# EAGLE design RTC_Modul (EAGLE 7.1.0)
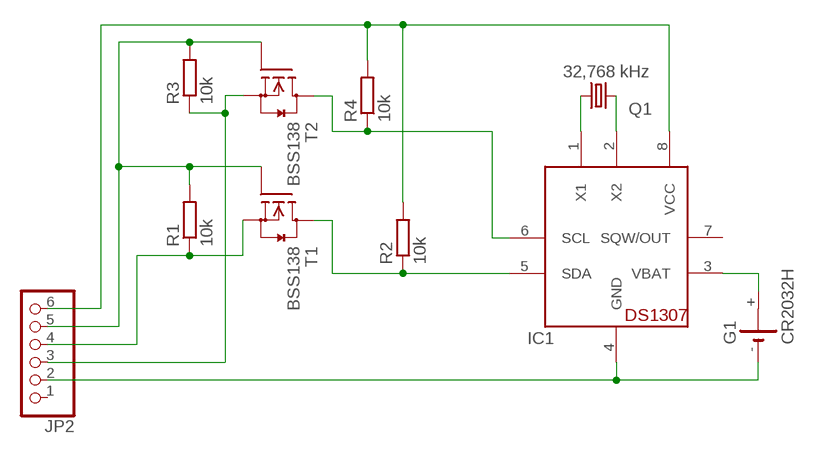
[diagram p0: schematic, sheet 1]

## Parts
G1  CR2032H  [CR2032H]
IC1  DS1307  [DIL08]
JP2  PINHD-1X6/90  [1X06/90]
Q1  32,768 kHz  CRYSTALTC26H  [TC26H]
R1  10k  R-EU_M1206  [M1206]
R2  10k  R-EU_M1206  [M1206]
R3  10k  R-EU_M1206  [M1206]
R4  10k  R-EU_M1206  [M1206]
T1  BSS138  [SOT23]
T2  BSS138  [SOT23]

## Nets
GND: G1.- IC1.4(GND) JP2.2
N$1: IC1.1(X1) Q1.1
N$2: IC1.2(X2) Q1.2
N$3: JP2.4 R1.1 T1.2(S)
N$5: G1.+ IC1.3(VBAT)
N$7: IC1.5(SDA) R2.1 T1.3(D)
N$9: JP2.3 R3.1 T2.2(S)
N$10: JP2.5 R1.2 R3.2 T1.1(G) T2.1(G)
N$11: IC1.6(SCL) R4.1 T2.3(D)
VCC: IC1.8(VCC) JP2.6 R2.2 R4.2
Unconnected: G1.+@1(+) IC1.7(SQW/OUT) JP2.1

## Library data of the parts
G1 = battery:CR2032H: LI BATTERY Varta
IC1 = adafruit:DS1307: DS1307 Real time clock (RTC) with battery backup ability. Talk to it via i2c
JP2 = pinhead:PINHD-1X6: PIN HEADER
Q1 = crystal:CRYSTAL: CRYSTAL; OC_FARNELL: unknown; OC_NEWARK: unknown
R1-R4 = rcl:R-EU_: RESISTOR, European symbol
T1 T2 = m-pad-2.1:BSS138: Fairchild Semiconductors BSS138 N-Channel Logic Level Enhancement Mode Field Effect Transistor General Description: These N-Channel enhancement mode field effect transistors are produced using Fairchild's proprietary, high cell density, DMOS technology. These products have been designed to minimize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

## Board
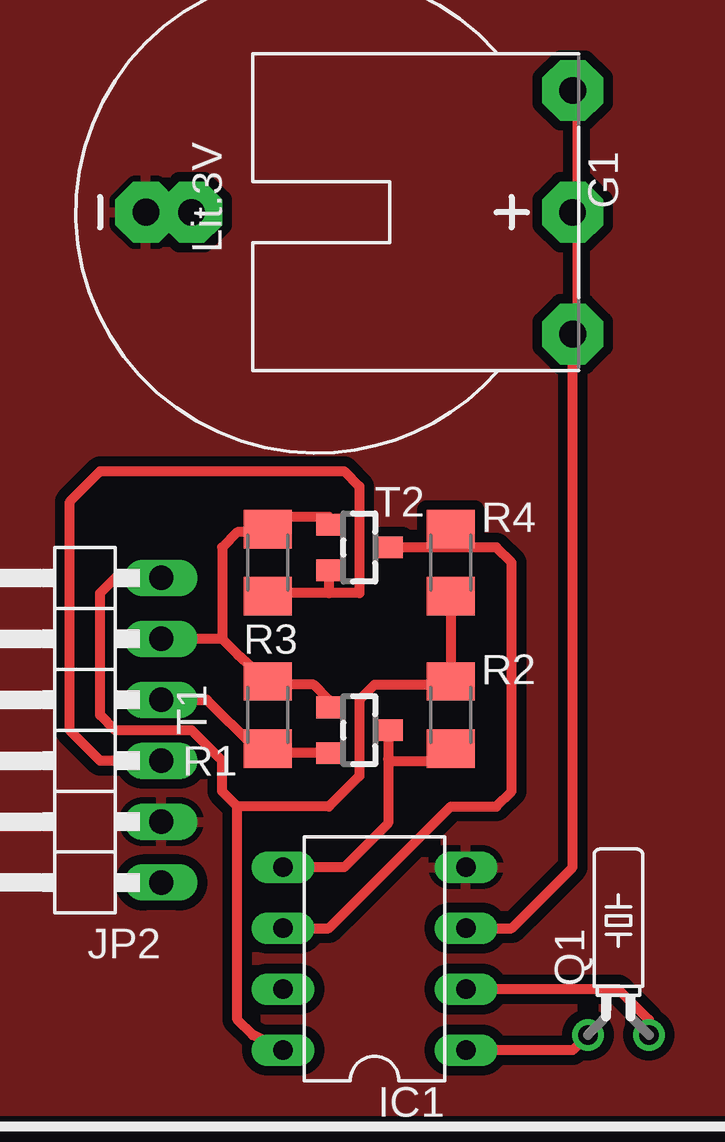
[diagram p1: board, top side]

No outline drawn. Coordinates in mm, seen from the top.
Copper layers (1*16): Top 0.035mm / dielectric 1.5mm / Bottom 0.035mm
Design rules "default": minimum track width 10mil, minimum drill 24mil, track to track 8mil, track to pad 8mil, pad to pad 8mil, via to via 8mil, smd to smd 8mil, copper to edge 40mil, drill to drill 8mil, minimum pad ring 10mil, minimum via ring 8mil, stop-mask expansion 4mil, vias tented up to drill 0mil, thermal gap 10mil

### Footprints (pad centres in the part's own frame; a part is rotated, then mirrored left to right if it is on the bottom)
CR2032H = drill 1.118 pad 2.54 octagon: + 5.08,10.795; +@1 -5.08,10.795; - 0,-6.985
DIL08 = drill 0.813 long: 1 -3.81,-3.81; 2 -1.27,-3.81; 3 1.27,-3.81; 4 3.81,-3.81; 5 3.81,3.81; 6 1.27,3.81; 7 -1.27,3.81; 8 -3.81,3.81
1X06/90 = drill 1.016 long: 1 -6.35,-3.81; 2 -3.81,-3.81; 3 -1.27,-3.81; 4 1.27,-3.81; 5 3.81,-3.81; 6 6.35,-3.81
TC26H = drill 0.813: 1 -1.27,0; 2 1.27,0
M1206 = smd 1.6 x 2: 1 -1.4,0; 2 1.4,0
SOT23 = smd 0.9 x 1.2: 1 -0.95,-1.2; 2 0.95,-1.2; 3 0,1.2

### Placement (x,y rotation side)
G1  17.78,38.1 270 top
IC1  20.32,6.99 90 top
JP2  7.62,16.51 90 top
Q1  30.48,3.81 0 top
R1  15.88,17.14 90 top
R2  23.5,17.14 90 top
R3  15.88,23.5 90 top
R4  23.5,23.5 270 top
T1  19.68,16.51 270 top
T2  19.68,24.13 270 top

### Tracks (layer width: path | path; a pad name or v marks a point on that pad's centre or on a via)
GND
  pour Top (isolate 0.406): 0.64,50.8 34.92,50.8 34.92,0.64 0.64,0.64
N$1
  Top 0.406: Q1.1 28.57,3.17 IC1.1
N$2
  Top 0.406: Q1.2 31.75,4.45 30.48,5.71 IC1.2
N$3
  Top 0.406: T1.2 16.2,15.56 15.88,15.24 R1.1 15.24,15.88 13.34,17.78 JP2.4
N$4  (via drill 1.1 pad 2.54)
  other vias: 28.57,38.1
N$5
  Top 0.406: IC1.3 26.04,8.26 28.57,10.79 G1.+
N$6  (via drill 1.1 pad 2.54)
  other vias: 12.7,38.1
N$7
  Top 0.406: 20.89,15.31 20.89,12.63 19.05,10.79 IC1.5 | T1.3 20.89,15.31 | 20.89,15.31 20.95,15.24 22.54,15.24 R2.1
N$9
  Top 0.406: 18.41,23.11 T2.2 18.48,22.93 18.41,22.86 18.41,22.23 | 18.41,22.23 19.68,22.23 19.68,26.67 19.05,27.3 8.89,27.3 7.62,26.04 7.62,16.51 8.89,15.24 JP2.3 | 18.41,22.23 15.88,22.23 R3.1
N$10
  Top 0.406: 13.97,20.32 14.61,19.68 R1.2 16,18.41 17.78,18.41 18.41,17.78 18.41,17.46 T1.1 | 13.97,20.32 JP2.5 | T2.1 18.41,25.4 16.38,25.4 R3.2 15.88,24.77 | 15.55,24.45 15.88,24.77 | 15.88,24.77 14.61,24.77 13.97,24.13 13.97,20.32
N$11
  Top 0.406: 23.5,24.13 25.4,24.13 26.04,23.5 26.04,13.97 25.4,13.34 23.5,13.34 18.41,8.26 IC1.6 | 23.5,24.13 R4.1 | 23.5,24.13 T2.3
VCC
  Top 0.406: R4.2 R2.2 23.5,18.41 20.32,18.41 19.68,17.78 19.68,14.61 18.41,13.34 14.61,13.34 | IC1.8 15.24,3.81 14.61,4.45 14.61,13.34 | 14.61,13.34 13.97,13.97 13.97,15.24 12.7,16.51 9.53,16.51 8.89,17.14 8.89,22.23 9.53,22.86 JP2.6
(copper drawn outside any net)
  shapes: Top area x2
